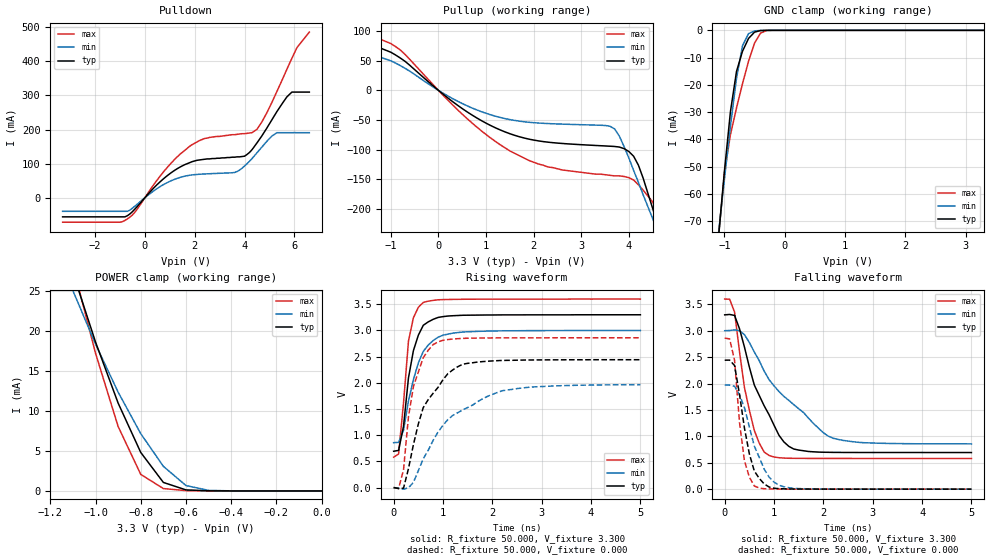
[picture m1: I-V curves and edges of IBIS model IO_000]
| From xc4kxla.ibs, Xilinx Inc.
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|   Model IO_000
[Model]   IO_000
Model_type   I/O
Polarity   Non-Inverting
Enable   Active-Low
Vinl =   0.800V
Vinh =   2.000V
Vmeas =   1.650V
Cref =  50.000pF
Rref =   1.000M
Vref =  0.000V
C_comp   7.300pF   5.500pF   8.800pF
[Temperature Range]   50.000   100.000   0.000
[Voltage Range]   3.300V   3.000V   3.600V
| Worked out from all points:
|   slope of the pulldown table from 0 to 0.495 V, typ, clamps not added: 12.8 ohm
|   slope of the pullup table from 0 to 0.495 V, typ, clamps not added: 16.3 ohm
|   GND clamp passes 1 mA (typ) near -0.52 V on its own axis
|   POWER clamp passes 1 mA (typ) near -0.69 V on its own axis
|   rising waveform, R_fixture 50.000, V_fixture 3.300: 20-80 % time 251ps typ, 353ps min, 189ps max; typ from 0.693 V to 3.3 V
|   rising waveform, R_fixture 50.000, V_fixture 0.000: 20-80 % time 599ps typ, 1.06ns min, 307ps max; typ from 0 V to 2.44 V
|   falling waveform, R_fixture 50.000, V_fixture 3.300: 20-80 % time 623ps typ, 1.14ns min, 333ps max; typ from 3.3 V to 0.694 V
|   falling waveform, R_fixture 50.000, V_fixture 0.000: 20-80 % time 284ps typ, 408ps min, 183ps max; typ from 2.44 V to 0.001 V
[Pulldown]
| voltage   I(typ)   I(min)   I(max)
-3.3V     -56.02mA   -39.74mA   -71.65mA
-900mV    -56.02mA   -39.74mA   -70.27mA
-400mV    -33.2mA    -24.66mA   -42.45mA
900mV     64.82mA    44.51mA    89.05mA
1.8V      103mA      66.09mA    151mA
3.6V      119mA      74.19mA    185mA
4V        122mA      93.03mA    188mA
4.5V      161mA      132mA      201mA
5.3V      253mA      191mA      312mA
5.7V      296mA      191mA      377mA
6.1V      310mA      191mA      440mA
6.6V      310mA      191mA      486mA
[Pullup]
| voltage   I(typ)   I(min)   I(max)
-3.3V     90.2mA     70.7mA     105mA
-1.9V     87mA       69.42mA    102mA
-1V       64.22mA    49.76mA    78.82mA
500mV     -30.67mA   -22.15mA   -40.1mA
1.5V      -72.97mA   -49.19mA   -102mA
2.3V      -87.2mA    -55.86mA   -129mA
3.6V      -94mA      -60.31mA   -143mA
3.8V      -95.43mA   -77.13mA   -144mA
4.1V      -111mA     -135mA     -151mA
4.5V      -199mA     -216mA     -188mA
4.7V      -250mA     -255mA     -227mA
6.6V      -645mA     -572mA     -737mA
[GND_clamp]
| voltage   I(typ)   I(min)   I(max)
-3.3V     -539mA     -461mA     -635mA
-1.1V     -76.29mA   -74.81mA   -76.3mA
-1V       -51.66mA   -54.6mA    -52.25mA
-900mV    -29.77mA   -35.09mA   -38.23mA
-800mV    -15.1mA    -17.65mA   -28.49mA
-700mV    -7.645mA   -5.66mA    -19.53mA
-600mV    -2.968mA   -1.205mA   -11.34mA
-500mV    -649uA     -202uA     -4.68mA
-400mV    -83.34uA   -28.89uA   -976uA
-300mV    -8.303uA   -3.567uA   -95.2uA
3.3V      90.24nA    487nA      4.544uA
[POWER_clamp]
| voltage   I(typ)   I(min)   I(max)
-3.3V     171mA      110mA      255mA
-1.1V     27.32mA    25.08mA    28.22mA
-1V       18.65mA    18.39mA    17.25mA
-900mV    11mA       12.37mA    8.069mA
-800mV    4.821mA    7.171mA    2.071mA
-700mV    1.064mA    3.083mA    296uA
-600mV    127uA      671uA      39.67uA
-500mV    14.7uA     70.21uA    9.223uA
0V        90.2nA     23.32nA    5.636uA
[Ramp]
| variable   typ   min   max
dV/dt_r   1.464/0.573n   1.178/1.039n   1.715/0.326n
dV/dt_f   1.563/0.595n   1.285/1.118n   1.810/0.337n
R_load = 50.000
[Rising Waveform]
R_fixture = 50.000
V_fixture = 3.300
V_fixture_min = 3.000
V_fixture_max = 3.600
L_fixture = 0.000H
C_fixture = 0.000F
| time   V(typ)   V(min)   V(max)
0s        693mV      856mV      580mV
100ps     709mV      863mV      640mV
200ps     1.17V      1.093V     1.613V
300ps     2.091V     1.651V     2.793V
400ps     2.613V     2.06V      3.241V
500ps     2.907V     2.377V     3.44V
600ps     3.097V     2.598V     3.534V
900ps     3.247V     2.87V      3.584V
1.3ns     3.284V     2.959V     3.593V
5ns       3.298V     2.998V     3.598V
[Rising Waveform]
R_fixture = 50.000
V_fixture = 0.000
V_fixture_min = 0.000
V_fixture_max = 0.000
L_fixture = 0.000H
C_fixture = 0.000F
| time   V(typ)   V(min)   V(max)
0s        0V         0V         0V
100ps     -18.86mV   -12.02mV   -18.64mV
200ps     -12.29mV   -30.91mV   339mV
300ps     360mV      -5.003mV   1.351V
400ps     817mV      98.42mV    1.924V
600ps     1.527V     550mV      2.478V
800ps     1.8V       902mV      2.729V
1.4ns     2.354V     1.482V     2.847V
2.2ns     2.426V     1.848V     2.857V
5ns       2.44V      1.964V     2.859V
[Falling Waveform]
R_fixture = 50.000
V_fixture = 3.300
V_fixture_min = 3.000
V_fixture_max = 3.600
L_fixture = 0.000H
C_fixture = 0.000F
| time   V(typ)   V(min)   V(max)
0s        3.3V       3V         3.599V
100ps     3.308V     3.004V     3.597V
200ps     3.289V     3.016V     3.353V
400ps     2.692V     2.925V     1.926V
600ps     1.972V     2.597V     1.113V
800ps     1.578V     2.234V     703mV
900ps     1.409V     2.074V     639mV
1.3ns     811mV      1.681V     586mV
2.2ns     697mV      964mV      583mV
5ns       694mV      858mV      582mV
[Falling Waveform]
R_fixture = 50.000
V_fixture = 0.000
V_fixture_min = 0.000
V_fixture_max = 0.000
L_fixture = 0.000H
C_fixture = 0.000F
| time   V(typ)   V(min)   V(max)
0s        2.442V     1.97V      2.861V
100ps     2.444V     1.97V      2.844V
200ps     2.341V     1.948V     2.439V
300ps     1.796V     1.788V     1.264V
400ps     1.159V     1.543V     539mV
500ps     668mV      1.178V     229mV
600ps     345mV      818mV      60.81mV
900ps     41.86mV    228mV      6.693mV
1.2ns     7.356mV    46.11mV    2.836mV
5ns       1.142mV    1.206mV    1.066mV
